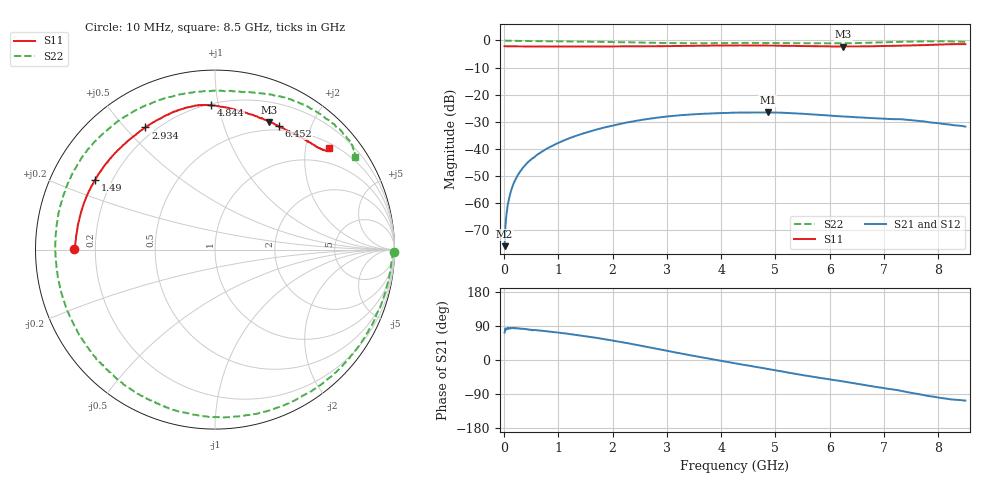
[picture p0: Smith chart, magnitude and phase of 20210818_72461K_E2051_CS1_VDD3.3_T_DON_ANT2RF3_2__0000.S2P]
!Agilent Technologies,E5071C,MY46417908,A.11.23
!Date: Wed Aug 18 14:29:09 2021
!Data & Calibration Information:
!Freq	S11:SOLT2(ON)	S21:SOLT2(ON)	S12:SOLT2(ON)	S22:SOLT2(ON)
!PortZ  Port1:50+j0  Port2:50+j0
!Above PortZ is port z conversion or system Z0 setting when saving the data.
!When reading, reference impedance value at option line is always used.
# Hz S dB R 50
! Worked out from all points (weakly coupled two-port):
!   1601 points, 10 MHz to 8.5 GHz, reference 50 ohm
!   highest |S21| = -26.54 dB at 4.86 GHz (marker M1); lowest = -75.8 dB at 10 MHz (marker M2)
!   lowest |S11| = -2.3 dB at 6.25 GHz (marker M3), VSWR 7.75, Z = 20.4 + j71.6 ohm
!   |S11| at or under -10 dB: nowhere
!   |S22| runs from -1.1 to 0.0 dB; largest |S21 - S12| = 0.00026
!   S11 on the Smith chart (normalised r, x): 10 MHz: 0.12, +0.00; 1.49 GHz: 0.14, +0.27; 2.934 GHz: 0.16, +0.57; 4.844 GHz: 0.21, +0.95; 6.452 GHz: 0.45, +1.55; 8.5 GHz: 0.60, +2.49
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1e7  -2.13 179.7  -75.82 72.6  -76.79 84.6  -0.01 -0.6
6.836875e7  -2.17 178.5  -60.43 82.6  -60.56 84.4  -0.11 -3.3
1.108188e8  -2.17 177.6  -56.64 83.6  -56.59 84.7  -0.13 -5.1
2.01025e8  -2.19 175.8  -51.65 83.4  -51.61 84.1  -0.15 -8.9
3.230688e8  -2.20 173.3  -47.57 82.5  -47.54 82.5  -0.19 -14.3
4.822562e8  -2.20 170.0  -44.16 79.9  -44.15 79.9  -0.26 -21.0
7.475688e8  -2.21 164.5  -40.35 76.4  -40.37 76.6  -0.30 -32.0
1.426769e9  -2.23 151.0  -34.48 64.3  -34.50 64.2  -0.45 -61.2
1.490444e9  -2.24 149.7  -34.10 62.9  -34.11 62.8  -0.45 -63.9
2.180256e9  -2.22 135.4  -30.58 46.9  -30.58 47.0  -0.64 -95.8
2.843538e9  -2.14 121.4  -28.40 28.7  -28.41 28.7  -0.90 -129.8
2.933744e9  -2.12 119.7  -28.21 26.3  -28.21 26.4  -0.93 -134.3
3.565188e9  -1.97 108.4  -27.16 8.9  -27.15 9.0  -1.03 -167.3
4.255e9  -1.85 98.8  -26.61 -8.6  -26.62 -8.5  -0.94 159.6
4.843994e9  -1.89 91.7  -26.55 -22.8  -26.56 -22.9  -0.93 134.7
4.859912e9  -1.89 91.5  -26.54 -23.2  -26.54 -23.2  -0.93 134.0
5.671769e9  -2.11 78.7  -27.26 -43.7  -27.26 -43.7  -1.04 103.5
6.25015e9  -2.25 66.9  -28.04 -56.7  -28.04 -56.8  -1.07 86.5
6.451788e9  -2.24 62.7  -28.26 -61.5  -28.27 -61.6  -1.00 81.0
7.088538e9  -2.02 50.6  -28.92 -76.3  -28.95 -76.5  -0.60 64.8
7.937538e9  -1.56 41.5  -30.38 -97.4  -30.36 -97.5  -0.31 43.3
8.5e9  -1.39 41.8  -31.75 -107.1  -31.74 -107.3  -0.57 33.6
